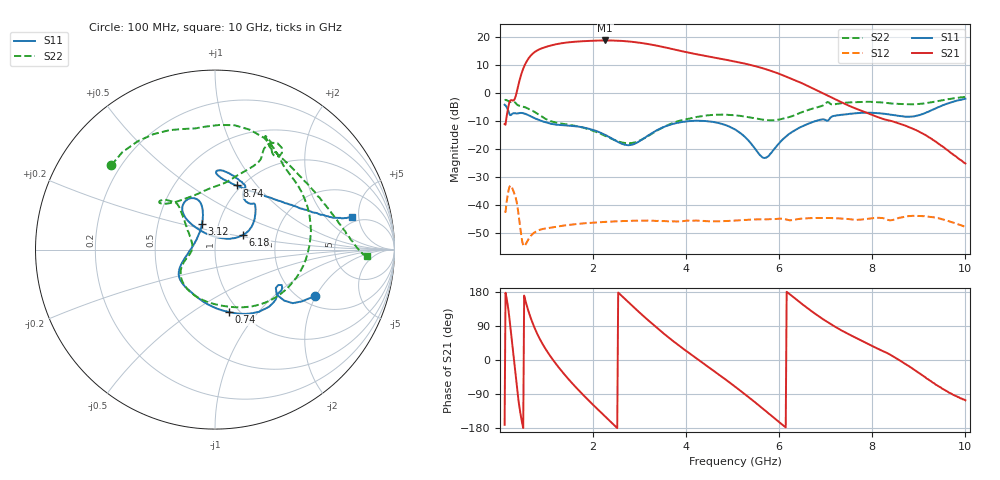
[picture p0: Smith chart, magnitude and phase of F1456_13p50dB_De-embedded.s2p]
! Integrated Device Technology
! Corporate Headquarters
! 6024 Silver Creek Valley Road
! San Jose, CA 95138  USA
! Phone:  1-408-284-8200
! Toll Free:  1-800-223-1366
! Webpage:  http://www.idt.com/
! Timing and RF Division
! 515 Groton Road, Suite 102
! Westford, MA 01886-6024
! Device:  F1456
! Description: 6-bit 0.5 dB Transmit Variable Gain Amplifier
! Frequency:  2100.0 -  2950.00 MHz
! Package:  6x6 mm Thin QFN Plastic Package: 28 pin
! State:  27
! Atten State:  13.5 dB
! Voltage:  +5.00 Volts
! Current:  216.997 mA
! Data:  The device was measured on a the F1455 evaluation board which has
!  individual transmission lines to the RF pins.  Data was collected
!  using a calibrated network analyzer.  The evaluation board was
!  de-embedded using a TRL calibration technique.
!  The reference plane is the edge of the package pin.
!  Pin  1 = CSb
!  Pin  2 = DATA
!  Pin  3 = CLK
!  Pin  4 = RSET
!  Pin  5 = GND
!  Pin  6 = RFIN  = Port 1
!  Pin  7 = GND
!  Pin  8 = NC
!  Pin  9 = NC
!  Pin 10 = NC
!  Pin 11 = NC
!  Pin 12 = NC
!  Pin 13 = NC
!  Pin 14 = /STBY
!  Pin 15 = GND
!  Pin 16 = RFOUT  = Port 2
!  Pin 17 = GND
!  Pin 18 = NC
!  Pin 19 = NC
!  Pin 20 = NC
!  Pin 21 = GND
!  Pin 22 = NC
!  Pin 23 = GND
!  Pin 24 = NC
!  Pin 25 = NC
!  Pin 26 = NC
!  Pin 27 = GND
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# GHz S dB R 50
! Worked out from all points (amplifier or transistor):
!   496 points, 100 MHz to 10 GHz, reference 50 ohm
!   highest |S21| = 18.6 dB at 2.26 GHz (marker M1)
!   |S21| within 3 dB of that: 868.6 MHz to 3.69 GHz (2.821 GHz wide, 124 % of centre)
!   unconditionally stable (mu >= 1): start of sweep to end of sweep
!   at 1.74 GHz: K = 11.41, MAG = 18.8 dB, |S12| = -46.5 dB
!   at 5.06 GHz: K = 20.83, MAG = 12.1 dB, |S12| = -45.4 dB
!   at 10 GHz: K = 240.80, MAG = -15.6 dB, |S12| = -47.6 dB
!   S11 on the Smith chart (normalised r, x): 100 MHz: 2.35, -1.96; 740 MHz: 0.90, -0.71; 3.12 GHz: 0.83, +0.24; 6.18 GHz: 1.35, +0.23; 8.74 GHz: 0.95, +0.79; 10 GHz: 4.30, +4.05
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0.1  -4.24 -25.1  -11.09 -171.0  -42.29 47.4  -2.56 140.9
0.32  -7.26 -32.3  -2.06 -20.7  -36.36 -145.2  -3.35 66.4
0.44  -7.15 -42.1  5.60 -141.4  -48.48 138.9  -4.66 38.6
0.58  -7.72 -59.5  11.36 142.0  -53.01 167.5  -5.42 6.9
0.74  -8.97 -77.7  14.43 85.9  -49.69 138.0  -6.74 -26.8
0.98  -10.47 -101.5  16.29 29.1  -48.26 93.3  -9.26 -69.0
1.2  -11.30 -118.6  17.26 -9.6  -47.71 68.7  -10.57 -96.7
1.5  -11.69 -135.5  18.01 -54.4  -46.91 43.7  -11.41 -124.8
1.76  -12.21 -145.5  18.34 -88.6  -46.47 26.5  -12.27 -141.1
2.26  -14.95 -162.9  18.63 -149.2  -45.91 -1.1  -15.30 -161.8
2.64  -18.25 167.5  18.44 166.3  -45.63 -20.2  -17.73 -177.9
3.12  -15.92 116.8  17.52 111.9  -45.46 -44.0  -16.02 152.0
3.4  -13.09 107.9  16.67 82.0  -45.53 -57.0  -13.24 138.8
3.74  -10.96 107.9  15.44 48.1  -45.73 -71.3  -10.57 130.9
4.1  -10.01 114.7  14.12 15.3  -45.55 -86.5  -9.05 131.2
5.06  -13.11 133.2  11.09 -71.1  -45.41 -128.3  -8.00 139.7
5.66  -23.12 84.2  8.67 -129.6  -45.02 -160.3  -9.58 122.7
6.18  -15.03 27.6  5.54 178.1  -45.19 168.0  -8.75 84.9
6.7  -10.50 41.2  1.77 128.3  -44.55 141.2  -5.69 64.9
8.36  -7.67 87.7  -9.84 15.8  -45.30 70.2  -3.73 62.3
8.74  -8.47 71.3  -11.86 -13.0  -43.92 60.0  -4.06 49.0
10  -2.12 13.5  -25.13 -106.2  -47.65 -23.3  -1.46 -2.6
